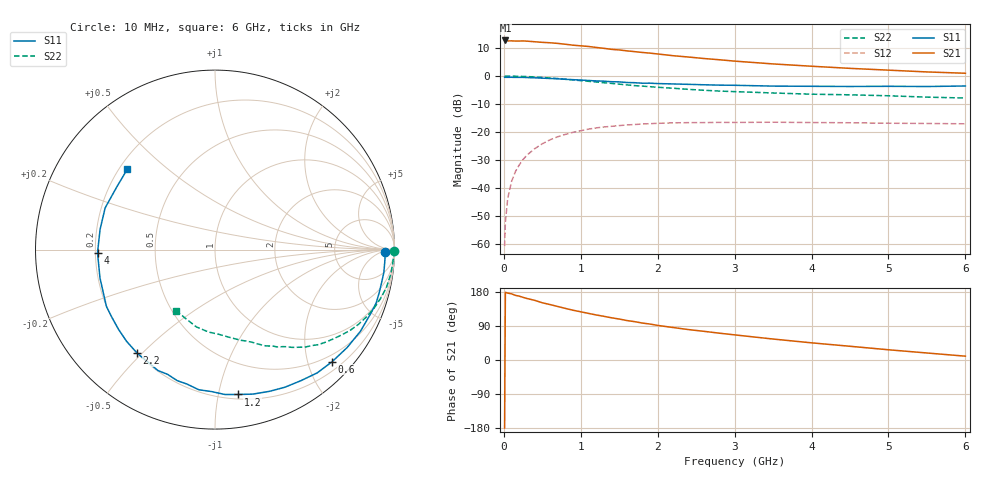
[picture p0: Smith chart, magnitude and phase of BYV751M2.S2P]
! SIEMENS Small Signal Semiconductors
! BFY420
! Si NPN RF SIEGET Grounded Emitter Transistor in MICRO-X
! VCE = 0.75 V  IC = 1.2 mA
! Common Emitter S-Parameters:  October  1996
# GHz  S  MA  R  50
!  f  S11  S21  S12  S22
! GHz  MAG  ANG  MAG  ANG  MAG  ANG  MAG  ANG
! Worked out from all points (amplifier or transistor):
!   36 points, 10 MHz to 6 GHz, reference 50 ohm
!   highest |S21| = 12.7 dB at 20 MHz (marker M1)
!   |S21| within 3 dB of that: start of sweep to 1.349 GHz
!   unconditionally stable (mu >= 1): 4.391 GHz to end of sweep
!   at 250 MHz: K = 0.05, MSG = 21.2 dB, |S12| = -29.9 dB
!   at 1.4 GHz: K = 0.26, MSG = 13.8 dB, |S12| = -18.0 dB
!   at 6 GHz: K = 1.32, MAG = 5.7 dB, |S12| = -17.1 dB
!   S11 on the Smith chart (normalised r, x): 10 MHz: 36, -11; 600 MHz: 0.36, -2.45; 1.2 GHz: 0.24, -1.15; 2.2 GHz: 0.20, -0.48; 4 GHz: 0.21, -0.01; 6 GHz: 0.23, +0.37
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0.01  0.9499 -0.9  4.326 -179.4  0.0009 99.3  0.9977 -0.5
0.02  0.9487 -1.6  4.333 178.6  0.0024 90.7  0.9933 -0.7
0.05  0.9484 -3.7  4.25 176.6  0.0064 89.0  0.9961 -2.1
0.1  0.9493 -7.6  4.26 174.6  0.0129 85.2  0.9934 -4.2
0.15  0.9464 -11.1  4.233 170.6  0.0194 82.2  0.9908 -6.3
0.25  0.9461 -18.3  4.251 165.3  0.032 77.8  0.9822 -10.4
0.4  0.9294 -29.3  4.109 157.5  0.0499 71.6  0.9617 -16.5
0.5  0.9164 -36.5  4.008 151.0  0.0613 67.2  0.9441 -20.3
0.6  0.9034 -43.7  3.94 146.3  0.0721 62.7  0.9231 -24.0
0.8  0.8735 -56.6  3.706 136.2  0.0902 54.6  0.8763 -31.0
0.9  0.8604 -62.9  3.565 131.3  0.0983 51.2  0.8512 -33.9
1.1  0.8323 -75.3  3.383 123.0  0.112 44.1  0.8045 -39.8
1.2  0.8178 -80.8  3.248 118.9  0.1178 40.9  0.7824 -42.6
1.6  0.7655 -101.7  2.822 104.1  0.133 30.1  0.6942 -51.7
2  0.7327 -119.4  2.482 91.3  0.1423 21.6  0.6291 -58.8
2.2  0.7217 -127.0  2.311 85.7  0.145 17.9  0.6051 -62.4
2.8  0.6871 -146.8  1.957 70.8  0.148 9.4  0.5381 -71.2
3.5  0.6601 -166.1  1.647 55.3  0.149 2.5  0.4972 -80.2
4  0.6548 -178.5  1.497 45.3  0.147 -1.5  0.473 -87.2
4.5  0.6501 170.0  1.372 36.2  0.1457 -5.0  0.4608 -94.4
5.5  0.6489 147.8  1.184 18.5  0.1414 -8.7  0.4189 -112.3
6  0.6633 137.4  1.121 10.1  0.1396 -9.5  0.4037 -122.4
